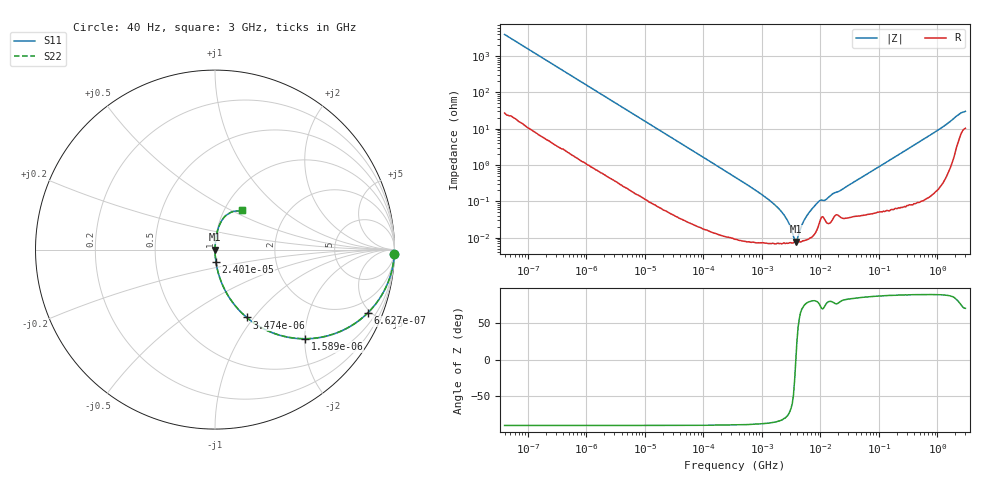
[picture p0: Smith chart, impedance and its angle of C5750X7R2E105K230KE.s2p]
! S-parameter Generated by TDK Corporation
! Copyright(C) 2015 TDK Corporation.
! All Rights Reserved.
! TDK P/N: C5750X7R2E105K230KE (Multilayer Ceramic Chip Capacitors)
! Property: C=1uF
! Size(LxWxT): 5.7x5x2.3mm, 0.224x0.197x0.091inches
! Model Type: s2p (Touchstone File Format Version 1.0)
! Frequency: DC=Yes Start=0.00004MHz Stop=3000MHz 396points Log-sweep
! Note: This model was converted from impedance.
! Model Generated on Jun. 23, 2015
! Hash(MD5):
! Port Assignments:
!  1 ---| |--- 2
! Applicable Conditions:
!  Temperature = 25 degC
!  DC Bias Voltage = 0 V
!  Small Signal Operation
! Terms and conditions regarding TDK Simulation Models
! (1)This simulation model is being provided solely for informational purposes. Please refer to the specifications of the products in terms of detailed characteristics of such products.
! (2)In no event shall TDK Corporation of any of its subsidiaries be liable for any loss or damage arising, directly or indirectly,
!  From any information contained in this simulation model, including, but not limited to loss or damages arising from any inaccuracies, omissions or errors in connection with such information.
! (3)Any and all copyrights on this simulation model are owned by TDK Corporation.
!  Duplication or redistribution of this simulation model without prior written permission from TDK Corporation is prohibited.
! (4)This simulation model is subject to any modification or change without any prior notice.
! (5)Neither TDK Corporation nor any of its subsidiaries shall make any warranty, express or implied,
!  Including but not limited to the correctness, implied warranties of merchantability and fitness for a particular purpose with respect to this simulation models.
! (6)The use of this simulation model shall be deemed to have consented to the terms and conditions hereof.
# MHz S MA R 50
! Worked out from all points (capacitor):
!   395 points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, 40 Hz to 3 GHz, reference 50 ohm
!   read as one part in series: C = 1.02 uF near 41.88 Hz
!   lowest |Z| = 7.82 mohm at 3.793 MHz (marker M1)
!   series resonance near 3.801 MHz, so ESL is about 1.7 nH
!   S11 on the Smith chart (normalised r, x): 40 Hz: 2, -78; 662.7 Hz: 1.03, -4.79; 1.589 kHz: 1.01, -2.01; 3.474 kHz: 1.01, -0.92; 24.01 kHz: 1.00, -0.13; 3 GHz: 1.21, +0.57
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4e-05  0.9995 -1.5  0.02553 88.1  0.02553 88.1  0.9995 -1.5
0.0001912643  0.992 -6.9  0.1202 82.7  0.1202 82.7  0.992 -6.9
0.000662667  0.9206 -22.6  0.3843 67.0  0.3843 67.0  0.9206 -22.6
0.000834128  0.883 -27.6  0.4636 62.0  0.4636 62.0  0.883 -27.6
0.001588756  0.7058 -44.7  0.7036 44.9  0.7036 44.9  0.7058 -44.7
0.003474114  0.4172 -64.9  0.9059 24.7  0.9059 24.7  0.4172 -64.9
0.01739424  0.09229 -84.3  0.9951 5.3  0.9951 5.3  0.09229 -84.3
0.02400588  0.06713 -85.7  0.9972 3.8  0.9972 3.8  0.06713 -85.7
0.3464102  0.004688 -88.6  0.9999 0.3  0.9999 0.3  0.004688 -88.6
1.901634  0.000652 -83.8  0.9999 0.0  0.9999 0.0  0.000652 -83.8
2.624455  0.000333 -77.6  0.9999 0.0  0.9999 0.0  0.000333 -77.6
3.013016  0.0002175 -70.2  0.9999 0.0  0.9999 0.0  0.0002175 -70.2
3.459106  0.0001096 -48.1  0.9999 0.0  0.9999 0.0  0.0001096 -48.1
3.792615  7.821e-05 -1.3  0.9999 0.0  0.9999 0.0  7.821e-05 -1.3
4.15828  0.0001102 44.8  0.9999 -0.0  0.9999 -0.0  0.0001102 44.8
5.234209  0.0002985 73.8  0.9999 -0.0  0.9999 -0.0  0.0002985 73.8
7.22376  0.0006308 80.3  0.9999 -0.0  0.9999 -0.0  0.0006308 80.3
9.521122  0.001026 76.0  0.9998 -0.1  0.9998 -0.1  0.001026 76.0
11.98465  0.00108 73.7  0.9997 -0.1  0.9997 -0.1  0.00108 73.7
150.6385  0.01347 86.9  0.9994 -0.8  0.9994 -0.8  0.01347 86.9
1371.938  0.125 80.9  0.9879 -7.2  0.9879 -7.2  0.125 80.9
3000  0.2641 55.7  0.8786 -14.4  0.8786 -14.4  0.2641 55.7
